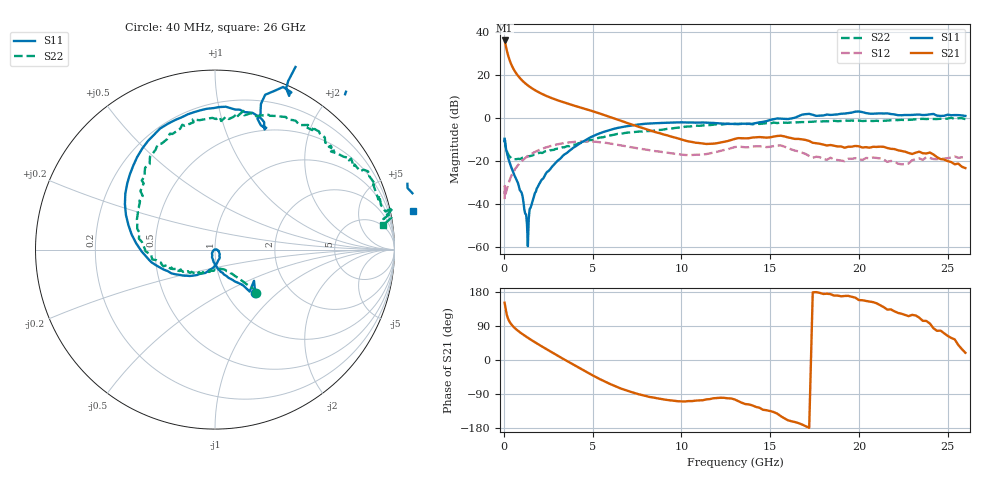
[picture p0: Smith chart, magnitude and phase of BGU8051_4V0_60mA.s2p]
! BGU8051_4V0_60mA
! Date/time Tue Jun 16 11:13:39 2015
! VAR V_out= 4.0000
! VAR I_out= 59.9800
! VAR V_in= 6.4380
! VAR I_in= 0.8333
# MHz S MA R 50
!  Freq-MHz  S11-mag  S11-arg  S21-mag  S21-arg  S12-mag  S12-arg  S22-mag  S22-arg
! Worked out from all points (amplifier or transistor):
!   197 points, 40 MHz to 26 GHz, reference 50 ohm
!   highest |S21| = 36.2 dB at 40 MHz (marker M1)
!   |S21| within 3 dB of that: start of sweep to 119.3 MHz
!   unconditionally stable (mu >= 1): 315.3 MHz to 13.18 GHz; 13.54 GHz to 13.71 GHz
!   at 800 MHz: K = 1.02, MAG = 19.9 dB, |S12| = -21.9 dB
!   at 6.4 GHz: K = 1.30, MAG = 2.6 dB, |S12| = -12.4 dB
!   at 26 GHz: K = -0.60, MSG = -2.6 dB, |S12| = -18.1 dB
!   lowest NFmin = 0.41 dB at 400 MHz
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40  0.3303 -47.2  64.83 151.0  0.01291 33.4  0.3357 -46.6
60  0.3031 -50.5  59.75 144.9  0.01989 28.8  0.2898 -46.4
80  0.2416 -53.1  54.39 138.8  0.01591 40.1  0.2421 -48.4
120  0.1929 -60.2  45.77 128.1  0.01881 47.4  0.1997 -51.3
160  0.1611 -66.3  38.62 119.9  0.02144 51.8  0.1745 -53.9
200  0.1363 -71.8  33.06 113.6  0.02436 56.2  0.1563 -56.9
260  0.1119 -80.4  26.98 106.3  0.03 59.6  0.1383 -60.3
320  0.09154 -85.3  22.63 100.9  0.03564 61.0  0.1275 -63.2
400  0.07385 -92.9  18.53 95.2  0.04317 62.9  0.1198 -66.6
500  0.05809 -99.9  15.08 89.6  0.05246 63.3  0.1138 -72.6
700  0.0372 -113.7  10.97 80.7  0.07134 61.3  0.1104 -80.5
900  0.02077 -132.9  8.61 73.2  0.08993 58.3  0.1109 -89.8
1350  0.00103 87.7  5.792 58.7  0.1297 49.8  0.1286 -104.8
1550  0.009341 5.8  5.059 52.6  0.1465 45.6  0.1324 -111.0
2700  0.07241 -79.5  2.923 20.4  0.2277 20.0  0.18 -136.6
4400  0.2775 -151.7  1.723 -25.1  0.2854 -18.9  0.2669 -156.3
6400  0.5895 147.9  0.929 -71.7  0.2399 -57.9  0.4289 171.7
8800  0.7687 101.4  0.4421 -102.3  0.1652 -77.6  0.5295 141.3
13200  0.7242 67.6  0.3418 -108.5  0.217 -91.5  0.7324 92.3
17400  1.197 49.0  0.2661 178.6  0.1186 -154.7  0.8239 64.3
21800  1.245 23.3  0.1923 133.5  0.1004 -166.9  0.8845 35.8
26000  1.125 11.1  0.06829 19.1  0.1249 176.7  0.9451 8.2
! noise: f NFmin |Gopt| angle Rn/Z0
400  0.4114  0.0091  252.1  0.0514
550  0.4161  0.02598  189.8  0.0503
950  0.4418  0.07759  179.7  0.0482
1250  0.4737  0.109  180.9  0.0476
1600  0.5245  0.1388  184.1  0.0481
1900  0.5798  0.1599  187.6  0.0496
2250  0.6579  0.1811  192.4  0.0528
2600  0.7506  0.2002  197.6  0.0576
3300  0.9802  0.2392  208.2  0.0725
4000  1.268  0.2864  217.2  0.0953
